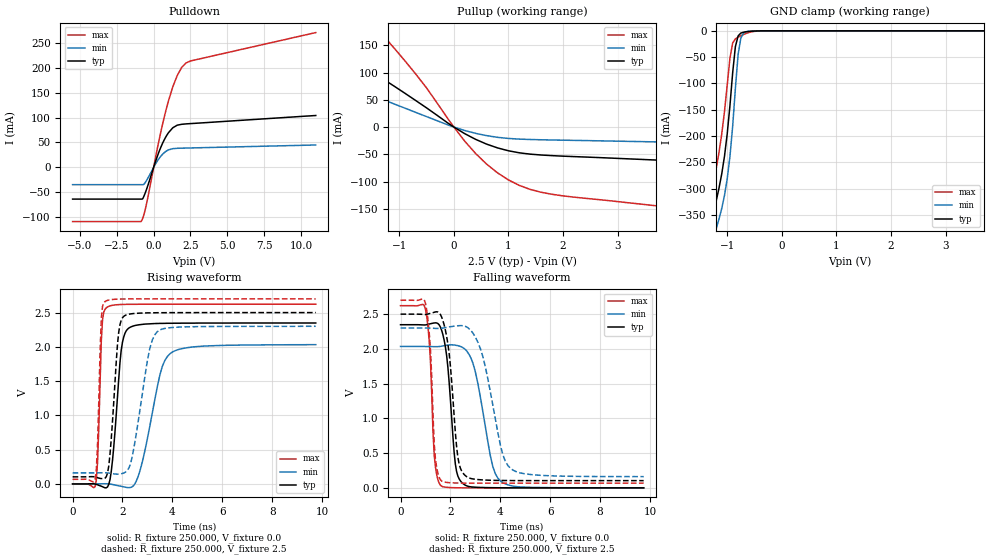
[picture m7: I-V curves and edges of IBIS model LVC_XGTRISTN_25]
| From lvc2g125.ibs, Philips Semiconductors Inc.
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|   Model LVC_XGTRISTN_25
[Model]   LVC_XGTRISTN_25
Model_type   3-state
Polarity   Non-Inverting
Enable   Active-Low
Vmeas =  1.25V
Cref  =  30.0pF
Rref  =  0.5k
Vref  =  0.0V
C_comp   3.90pF   2.97pF   5.09pF
[Model Spec]
| Note: The input and output voltage ratings may be exceeded if the input and
|   output current ratings are observed (please refer to the data sheet)
|   Subparameter   typ   min   max
| Timing Thresholds
Vmeas   1.25   1.15   1.35
|Ambient temperature:   25   85   -40
[Temperature Range]   30   90   -35
[Voltage Range]   2.5V   2.3V   2.7V
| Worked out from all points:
|   slope of the pulldown table from 0 to 0.375 V, typ, clamps not added: 11.7 ohm
|   slope of the pullup table from 0 to 0.375 V, typ, clamps not added: 17.6 ohm
|   GND clamp passes 1 mA (typ) near -0.58 V on its own axis
|   rising waveform, R_fixture 250.000, V_fixture 0.0: 20-80 % time 297ps typ, 677ps min, 132ps max; typ from 0 V to 2.35 V
|   rising waveform, R_fixture 250.000, V_fixture 2.5: 20-80 % time 263ps typ, 551ps min, 125ps max; typ from 0.104 V to 2.5 V
|   falling waveform, R_fixture 250.000, V_fixture 0.0: 20-80 % time 304ps typ, 612ps min, 190ps max; typ from 2.35 V to 0 V
|   falling waveform, R_fixture 250.000, V_fixture 2.5: 20-80 % time 333ps typ, 710ps min, 197ps max; typ from 2.5 V to 0.104 V
|Process Range   nominal   slow   fast
[Pulldown]
| voltage   I(typ)   I(min)   I(max)
-5.5V     -63.99mA   -34.95mA   -109.2mA
-850mV    -63.99mA   -34.95mA   -109.2mA
-750mV    -63.57mA   -34.95mA   -103.4mA
-500mV    -45.76mA   -27.27mA   -75.73mA
400mV     34.05mA    19.16mA    59.41mA
700mV     54.21mA    29mA       98.79mA
1V        69.46mA    35mA       133.2mA
1.3V      79.62mA    37.55mA    162.1mA
1.6V      84.79mA    38.24mA    184.8mA
1.9V      86.59mA    38.54mA    200.9mA
2.2V      87.38mA    38.76mA    210.1mA
11V       104.3mA    44.93mA    271.2mA
[Pullup]
| voltage   I(typ)   I(min)   I(max)
-8.7V     282.9mA    126.7mA    774.1mA
-3.9V     229.5mA    126.7mA    430.1mA
-3.1V     190.5mA    109.3mA    364.9mA
-2.5V     162.5mA    91.01mA    304.5mA
-1.5V     101.1mA    57.93mA    190.5mA
-900mV    62.23mA    34.84mA    121.9mA
400mV     -22.59mA   -11.55mA   -48.63mA
800mV     -38.21mA   -18.79mA   -83.99mA
1.2V      -47.23mA   -22.08mA   -107mA
2.2V      -54.16mA   -24.4mA    -128.5mA
7.2V      -75.58mA   -33.77mA   -182.2mA
8.2V      -79.9mA    -35.65mA   -193.1mA
[GND_clamp]
| voltage   I(typ)   I(min)   I(max)
-5.5V     -4.549A    -4.577A    -4.533A
-1.35V    -431.2mA   -478.5mA   -376.2mA
-1.3V     -387mA     -434.9mA   -331.3mA
-1.2V     -322.7mA   -375.8mA   -261mA
-1.05V    -238.7mA   -313.3mA   -153.9mA
-950mV    -142.4mA   -239.2mA   -52.24mA
-900mV    -79.99mA   -181.7mA   -23.3mA
-850mV    -30.03mA   -109.5mA   -15.34mA
-800mV    -9.691mA   -44.99mA   -11.97mA
-750mV    -4.311mA   -13.93mA   -9.302mA
-700mV    -2.635mA   -4.184mA   -6.926mA
5.5V      274pA      2.383nA    27.39pA
[Ramp]
| variable   typ   min   max
dV/dt_r   1.409V/296.710ps   1.219V/677.260ps   1.573V/131.827ps
dV/dt_f   1.438V/333.127ps   1.283V/710.406ps   1.579V/197.146ps
R_load = 250.000
[Rising Waveform]
R_fixture   = 250.000
V_fixture   = 0.0
V_fixture_min = 0.0
V_fixture_max = 0.0
| time   V(typ)   V(min)   V(max)
0s        13.84pV    664.6pV    -7.153pV
950ps     -6.257mV   512.9uV    53.4mV
1.2ns     -40.55mV   2.524mV    2.398V
1.35ns    -56.99mV   2.891mV    2.569V
1.6ns     344.1mV    -7.905mV   2.606V
1.95ns    1.955V     -34.35mV   2.618V
2.25ns    2.273V     -54.11mV   2.62V
2.7ns     2.324V     192.7mV    2.622V
3.9ns     2.344V     1.898V     2.622V
9.75ns    2.348V     2.032V     2.622V
[Rising Waveform]
R_fixture   = 250.000
V_fixture   = 2.5
V_fixture_min = 2.3
V_fixture_max = 2.7
| time   V(typ)   V(min)   V(max)
0s        103.8mV    161.3mV    67.5mV
900ps     101.5mV    161.7mV    65.07mV
1ns       90.86mV    162.2mV    579mV
1.15ns    78.52mV    162.8mV    2.413V
1.3ns     84.07mV    162.3mV    2.661V
1.5ns     435.7mV    156mV      2.687V
1.85ns    2.216V     143.5mV    2.697V
2.05ns    2.445V     159.2mV    2.698V
3.4ns     2.498V     2.223V     2.7V
9.75ns    2.5V       2.3V       2.7V
[Falling Waveform]
R_fixture   = 250.000
V_fixture   = 0.0
V_fixture_min = 0.0
V_fixture_max = 0.0
| time   V(typ)   V(min)   V(max)
0s        2.348V     2.035V     2.622V
1ns       2.345V     2.034V     2.572V
1.2ns     2.362V     2.033V     1.825V
1.35ns    2.373V     2.032V     475.3mV
1.65ns    2.267V     2.039V     23.01mV
1.9ns     1.733V     2.055V     6.398mV
2.2ns     338.8mV    2.053V     1.657mV
2.5ns     62.54mV    2.018V     396uV
4ns       1.035mV    101.5mV    -13.36uV
9.75ns    -4.74uV    -29.28uV   -1.14nV
[Falling Waveform]
R_fixture   = 250.000
V_fixture   = 2.5
V_fixture_min = 2.3
V_fixture_max = 2.7
| time   V(typ)   V(min)   V(max)
0s        2.5V       2.3V       2.7V
1ns       2.495V     2.3V       2.656V
1.2ns     2.512V     2.298V     1.988V
1.4ns     2.532V     2.295V     414.7mV
1.65ns    2.457V     2.297V     97.4mV
1.95ns    1.933V     2.316V     74.38mV
2.3ns     439.2mV    2.333V     69.02mV
2.6ns     175.6mV    2.324V     67.9mV
4.4ns     104.9mV    284.1mV    67.49mV
9.75ns    103.8mV    161.5mV    67.5mV
